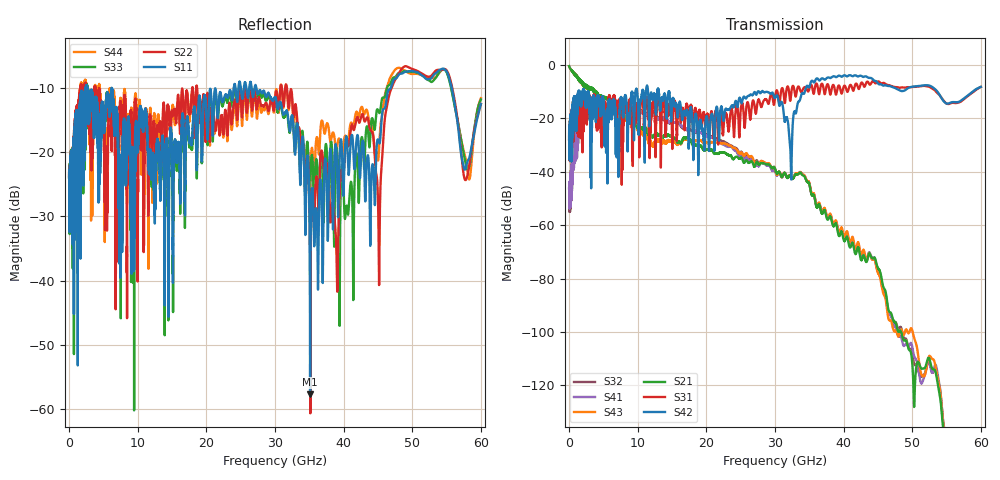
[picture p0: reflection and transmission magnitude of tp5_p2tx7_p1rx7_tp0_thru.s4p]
! 100G CR Analysis
! File: tp5_p2tx7_p1rx7_tp0_thru
! Description: 2m Cu Cable, OSFP, TP0-TP5
! Port Mapping
! Port1 -- P1RX7N
! Port2 -- P2TX7N
! Port3 -- P1RX7P
! Port4 -- P2TX7P
# GHz S MA R 50.00
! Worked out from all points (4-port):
!   6000 points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, 10 MHz to 60 GHz, reference 50 ohm
!   strongest paths, dB at 10 MHz, 15.01 GHz, 30.01 GHz, 45.01 GHz, 60 GHz:
!     S42: -27.9, -14.7, -12.4, -6.9, -8.2
!     S31: -27.9, -26.0, -12.2, -6.2, -8.2
!     S21: -0.5, -26.9, -39.0, -76.2, -177.5
!     S43: -0.5, -28.6, -39.1, -77.9, -175.6
!     S41: -45.9, -21.2, -39.8, -76.4, -177.1
!     S32: -46.3, -21.2, -38.9, -77.4, -172.9
!   lowest |S11| = -57.7 dB at 35.12 GHz (marker M1), VSWR 1.00, Z = 50 - j0.126 ohm
!   |S11| at or under -10 dB: 6.211 GHz to 24 GHz (17.79 GHz wide, 118 % of centre); 27.29 GHz to 46.86 GHz (19.58 GHz wide, 52.8 % of centre); 55.75 GHz to end of sweep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
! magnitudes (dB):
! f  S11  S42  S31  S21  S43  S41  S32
! 10 MHz  -24.0  -27.9  -27.9  -0.5  -0.5  -45.9  -46.3
! 6.87 GHz  -14.0  -32.4  -19.5  -17.1  -17.2  -13.8  -13.6
! 28.86 GHz  -11.1  -10.1  -13.5  -37.3  -37.0  -37.8  -37.1
! 32.27 GHz  -16.1  -33.3  -13.0  -41.7  -41.6  -41.7  -41.6
! 35.12 GHz  -57.7  -7.3  -7.9  -46.1  -45.6  -45.8  -46.0
! 45.56 GHz  -14.5  -7.4  -6.9  -80.4  -83.0  -81.1  -81.9
! 60 GHz  -12.5  -8.2  -8.2  -177.5  -175.6  -177.1  -172.9
